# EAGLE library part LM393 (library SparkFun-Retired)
Low-voltage comparator Prototype: IC-09375
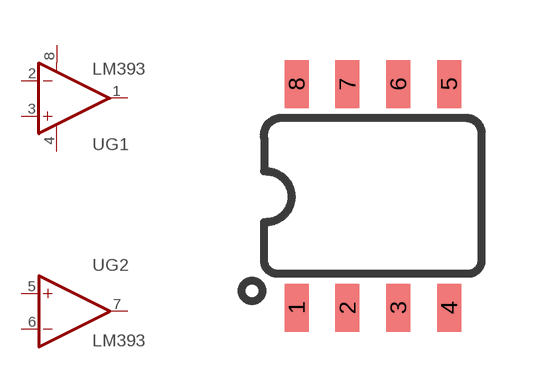
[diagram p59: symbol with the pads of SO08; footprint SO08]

Designator prefix -; gates G1=OP-AMP+- G2=OP-AMP

## LM393  [SO08]
1  G1:OUT  out
2  G1:-IN  in
3  G1:+IN  in
4  G1:V-  pwr
5  G2:+IN  in
6  G2:-IN  in
7  G2:OUT  out
8  G1:V+  pwr

## Footprint SO08 (pad centres in mm)
SOIC, 0.15 inch width
smd 0.6 x 1.2: 1 -1.905,-2.8; 2 -0.635,-2.8; 3 0.635,-2.8; 4 1.905,-2.8; 5 1.905,2.8; 6 0.635,2.8; 7 -0.635,2.8; 8 -1.905,2.8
